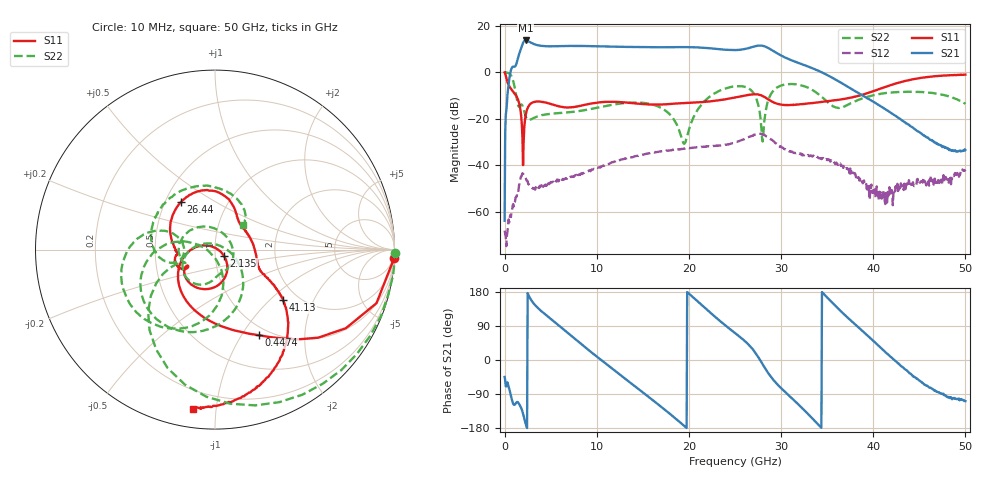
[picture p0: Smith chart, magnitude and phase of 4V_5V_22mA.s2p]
! MARKI MICROWAVE INC.
! Date:  1/07/2020
! Model Number:  APM-6849CH
! Description:  2-port Small Signal S-parameter data for APM-6849CH
! Frequency Range:  10 MHz to 50 GHz
! Port Configuration:  PORT 1: Input
!  PORT 2: Output
! Bias Condition: Vc = +4V, Vb = +5V
! APM-6849CH s2p files are only valid for small signal conditions (below -5 dBm input power)
!S2P File: Measurements: Mag<S11> Ang<S11>, Mag<S21> Ang<S21>, Mag<S12> Ang<S12>, Mag<S22> Ang<S22>!row 1
# Hz S  dB  R 50
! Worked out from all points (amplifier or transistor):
!   801 points, 10 MHz to 50 GHz, reference 50 ohm
!   highest |S21| = 13.8 dB at 2.322 GHz (marker M1)
!   |S21| within 3 dB of that: 1.832 GHz to 20.96 GHz (19.13 GHz wide, 168 % of centre)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
!   unconditionally stable (mu >= 1): 106 MHz to end of sweep
!   at 8.321 GHz: K = 19.00, MAG = 11.7 dB, |S12| = -43.5 dB
!   at 25 GHz: K = 3.74, MAG = 11.3 dB, |S12| = -30.2 dB
!   at 50 GHz: K = 564.16, MAG = -26.3 dB, |S12| = -41.9 dB
!   S11 on the Smith chart (normalised r, x): 10 MHz: 1, -42; 447.4 MHz: 0.89, -1.19; 2.135 GHz: 1.10, -0.07; 26.44 GHz: 0.60, +0.36; 41.13 GHz: 1.67, -1.21; 50 GHz: 0.10, -0.87
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1e7  -0.00 -2.7  -63.94 -44.8  -68.23 116.1  0.04 -1.0
4.474125e8  -5.43 -63.0  -4.76 -70.5  -63.38 -5.7  -0.37 -51.2
1.5097e9  -12.25 -147.6  6.89 -113.0  -50.90 -77.3  -14.59 -157.0
2.134575e9  -24.44 -34.0  13.49 -153.9  -44.52 -148.8  -16.84 116.3
2.322038e9  -17.90 -57.3  13.76 -170.5  -45.79 -165.3  -19.27 79.2
3.071888e9  -12.93 -102.4  12.40 152.0  -49.77 178.9  -19.87 -5.8
4.571588e9  -13.10 -139.8  11.26 117.1  -48.84 174.0  -18.07 -51.3
8.383325e9  -14.25 -146.5  11.39 40.7  -43.76 129.3  -16.50 -86.0
1.175765e10  -12.65 -163.0  11.10 -24.3  -38.72 90.6  -13.91 -106.5
1.431964e10  -13.43 -172.7  10.91 -72.6  -36.04 53.6  -12.98 -131.4
1.669416e10  -13.87 -173.7  10.84 -117.7  -34.27 16.9  -14.75 -162.8
2.038092e10  -13.07 179.1  10.83 167.2  -32.43 -43.6  -20.49 -13.3
2.263048e10  -12.34 170.1  10.26 118.5  -31.69 -87.4  -9.40 -69.0
2.5005e10  -10.82 149.6  9.62 71.1  -30.23 -133.5  -6.01 -118.4
2.644221e10  -9.74 125.4  10.43 41.5  -28.00 -172.7  -6.80 -155.5
2.775445e10  -9.75 89.7  11.57 -1.0  -26.51 133.2  -19.18 163.8
2.906669e10  -12.66 59.5  9.44 -49.5  -29.29 78.6  -8.37 -96.7
3.094131e10  -14.11 35.9  5.57 -95.6  -34.00 35.1  -5.02 -145.5
3.337832e10  -13.23 3.1  1.80 -153.5  -36.30 -7.5  -7.54 169.9
4.112678e10  -6.54 -36.5  -15.40 25.7  -52.82 80.3  -9.05 174.4
4.168916e10  -5.78 -39.8  -16.82 12.9  -52.50 70.8  -8.76 167.9
5e10  -0.98 -97.8  -33.45 -108.4  -41.90 -75.6  -13.62 41.4
